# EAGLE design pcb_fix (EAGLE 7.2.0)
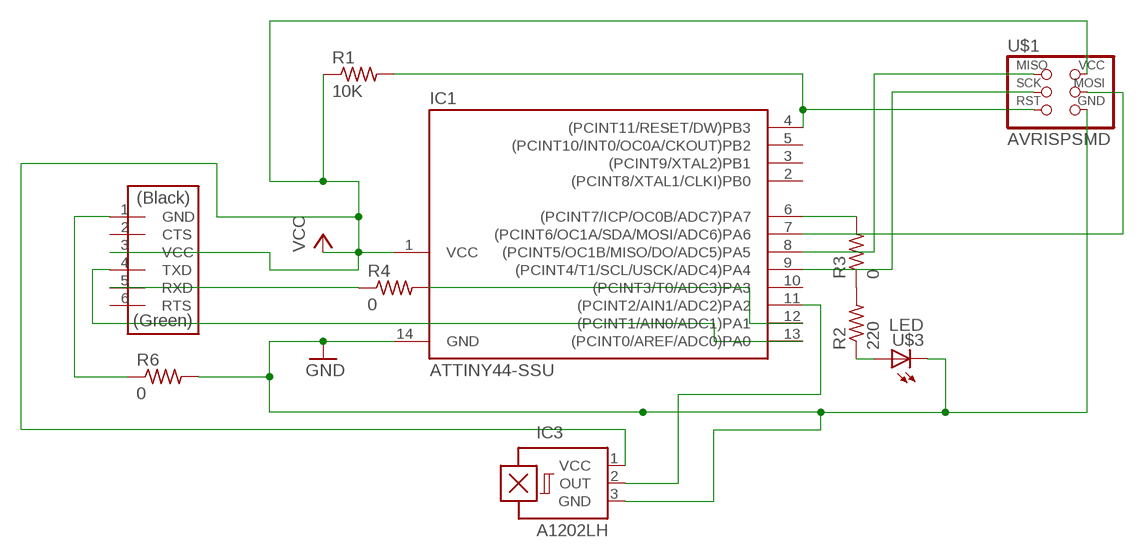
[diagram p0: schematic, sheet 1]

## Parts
IC1  ATTINY44-SSU  [SOIC14]
IC3  A1202LH  [SOT23-W]
R1  10K  RES-US1206  [R1206]
R2  220  RES-US1206FAB  [R1206FAB]
R3  0  RES-US1206FAB  [R1206FAB]
R4  0  RES-US1206FAB  [R1206FAB]
R6  0  RES-US1206FAB  [R1206FAB]
U$1  AVRISPSMD  [2X03SMD]
U$2  FTDI-SMD-HEADER  [1X06SMD]
U$3  LED  [LED1206]

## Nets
GND: IC1.14(GND) IC3.3(GND) R6.2 U$1.6(GND) U$3.2(C)
N$1: IC1.8((PCINT5/OC1B/MISO/DO/ADC5)PA5) U$1.1(MISO)
N$2: IC1.9((PCINT4/T1/SCL/USCK/ADC4)PA4) U$1.3(SCK)
N$3: IC1.4((PCINT11/RESET/DW)PB3) R1.2 U$1.5(RST)
N$4: R2.1 U$3.1(A)
N$5: IC1.6((PCINT7/ICP/OC0B/ADC7)PA7) R3.2
N$6: IC1.7((PCINT6/OC1A/SDA/MOSI/ADC6)PA6) U$1.4(MOSI)
N$7: R2.2 R3.1
N$8: IC1.12((PCINT1/AIN0/ADC1)PA1) R4.2
N$9: IC1.13((PCINT0/AREF/ADC0)PA0) U$2.4(TXD)
N$10: R4.1 U$2.5(RXD)
N$13: IC1.11((PCINT2/AIN1/ADC2)PA2) IC3.2(OUT)
N$14: R6.1 U$2.1(GND)
VCC: IC1.1(VCC) IC3.1(VCC) R1.1 U$1.2(VCC) U$2.3(VCC)
Unconnected: IC1.2((PCINT8/XTAL1/CLKI)PB0) IC1.3((PCINT9/XTAL2)PB1) IC1.5((PCINT10/INT0/OC0A/CKOUT)PB2) IC1.10((PCINT3/T0/ADC3)PA3) U$2.2(CTS) U$2.6(RTS)

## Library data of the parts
IC1 = fab:ATTINY44
IC3 = allegro:A12*?: Hall-effect bipolar switch Source: http://www.allegromicro.com/en/Products/Part_Numbers/1202/1202.pdf; OC_FARNELL: unknown; OC_NEWARK: unknown
R1-R4 R6 = fab:RES-US: Resistor (US Symbol)
U$1 = fab:AVRISP
U$2 = fab:FTDI-SMD-HEADER
U$3 = fab:LED: LED

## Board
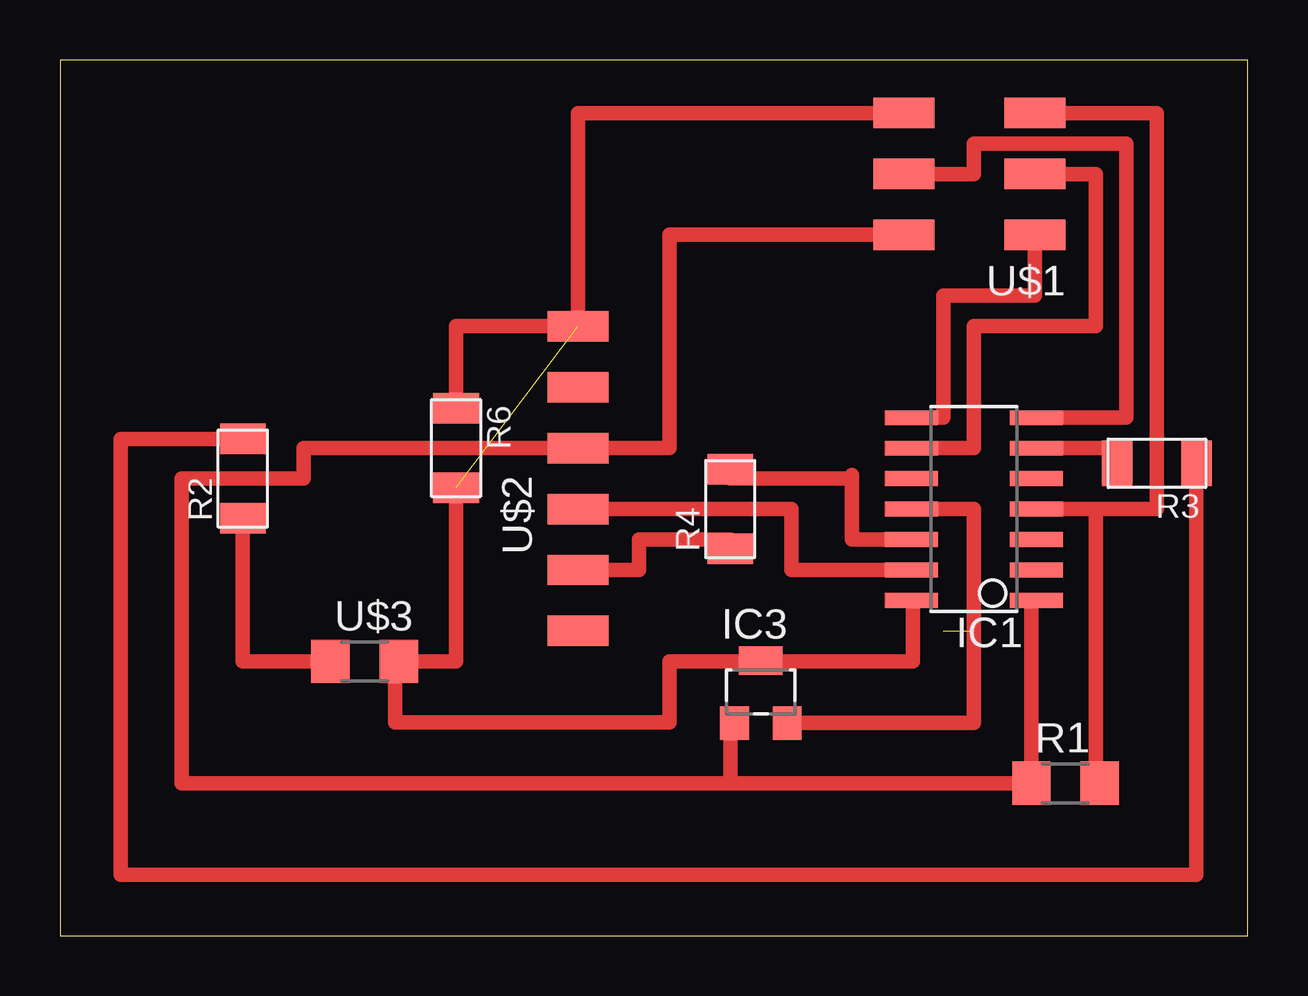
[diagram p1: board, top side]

Size 49.51 x 36.5 mm. Coordinates in mm from the lower left corner, seen from the top.
Outline: 0,0 49.51,0 49.51,36.5 0,36.5 0,0
Copper layers (1*16): Top 0.035mm / dielectric 1.5mm / Bottom 0.035mm
Design rules "default": minimum track width 10mil, minimum drill 24mil, track to track 8mil, track to pad 8mil, pad to pad 8mil, via to via 8mil, smd to smd 8mil, copper to edge 40mil, drill to drill 8mil, minimum pad ring 10mil, minimum via ring 8mil, stop-mask expansion 4mil, vias tented up to drill 0mil, thermal gap 10mil

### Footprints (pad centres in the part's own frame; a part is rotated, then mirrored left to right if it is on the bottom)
SOIC14 = smd 0.61 x 2.21: 1 -3.81,-2.603; 2 -2.54,-2.603; 3 -1.27,-2.603; 4 0,-2.603; 5 1.27,-2.603; 6 2.54,-2.603; 7 3.81,-2.603; 8 3.81,2.603; 9 2.54,2.603; 10 1.27,2.603; 11 0,2.603; 12 -1.27,2.603; 13 -2.54,2.603; 14 -3.81,2.603
SOT23-W = smd 1.2 x 1.4: 1 -1.1,-1.3; 2 1.1,-1.3 | smd 1.8 x 1.2: 3 0,1.3
R1206 = smd 1.6 x 1.803: 1 -1.422,0; 2 1.422,0
R1206FAB = smd 1.27 x 1.905: 1 -1.651,0; 2 1.651,0
2X03SMD = smd 2.54 x 1.27: 1 -2.54,2.54; 2 2.92,2.54; 3 -2.54,0; 4 2.92,0; 5 -2.54,-2.54; 6 2.92,-2.54
1X06SMD = smd 2.54 x 1.27: 1 0,6.35; 2 0,3.81; 3 0,1.27; 4 0,-1.27; 5 0,-3.81; 6 0,-6.35
LED1206 = smd 1.6 x 1.803: 1 -1.422,0; 2 1.422,0

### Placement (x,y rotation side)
IC1  38.1,17.78 90 top
IC3  29.21,10.16 0 top
R1  41.91,6.35 0 top
R2  7.62,19.05 90 top
R3  45.72,19.68 180 top
R4  27.94,17.78 90 top
R6  16.51,20.32 270 top
U$1  38.1,31.75 180 top
U$2  21.59,19.05 0 top
U$3  12.7,11.43 0 top

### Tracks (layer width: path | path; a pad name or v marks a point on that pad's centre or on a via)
GND  (1 unrouted)
  Top 0.406: U$3.2 13.97,11.43 | IC1.14 35.56,13.97 | 29.21,11.43 IC3.3
  Top 0.61: U$3.2 16.51,11.43 R6.2 | U$1.6 21.59,34.29 21.59,25.4 | 13.97,11.43 13.97,8.89 25.4,8.89 25.4,11.43 29.21,11.43 35.56,11.43 35.56,13.97
N$1
  Top 0.61: IC1.8 36.83,21.59 36.83,26.67 40.64,26.67 U$1.1
N$2
  Top 0.61: IC1.9 38.1,20.32 38.1,25.4 43.18,25.4 43.18,31.75 U$1.3
N$3
  Top 0.61: R1.2 43.18,6.35 43.18,17.78 | 43.18,17.78 IC1.4 | U$1.5 45.72,34.29 45.72,17.78 43.18,17.78
N$4
  Top 0.61: U$3.1 7.62,11.43 R2.1
N$5
  Top 0.61: IC1.6 44.07,20.32 R3.2
N$6
  Top 0.61: IC1.7 44.45,21.59 44.45,33.02 38.1,33.02 38.1,31.75 U$1.4
N$7
  Top 0.61: R2.2 2.54,20.7 2.54,2.54 47.37,2.54 R3.1
N$8
  Top 0.61: 33.02,19.2 33.02,19.05 | IC1.12 33.02,16.51 33.02,19.05 | 33.02,19.05 27.94,19.05 R4.2
N$9
  Top 0.61: U$2.4 30.48,17.78 30.48,15.24 IC1.13
N$10
  Top 0.61: U$2.5 24.13,15.24 24.13,16.51 27.94,16.51 R4.1
N$13  (1 unrouted)
  Top 0.61: IC1.11 38.1,17.78 38.1,12.7 38.1,8.86 IC3.2
N$14
  Top 0.61: R6.1 16.51,25.4 U$2.1
VCC
  Top 0.406: IC3.1 27.94,8.86
  Top 0.61: 27.94,6.35 5.08,6.35 5.08,19.05 10.16,19.05 10.16,20.32 U$2.3 25.4,20.32 25.4,29.21 U$1.2 | 27.94,6.35 R1.1 40.49,13.97 IC1.1 | 27.94,8.86 27.94,6.35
